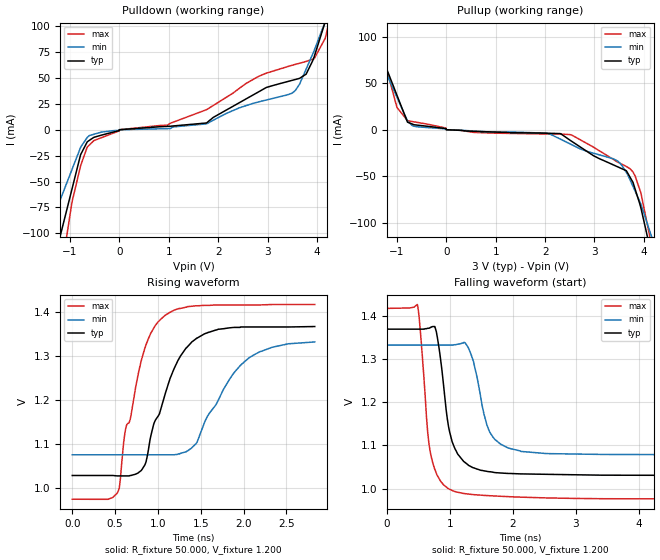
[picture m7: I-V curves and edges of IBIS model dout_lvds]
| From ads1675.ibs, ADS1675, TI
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|   dout_lvds Model
[Model]   dout_lvds
Model_type   Output
Polarity   Non-Inverting
Vmeas = 1.2
Vref = 1.2
Cref = 15pF
Rref = 50
|   typ   min   max
|   (nom PVT)   (Fast PVT)   (slow PVT)
|C_comp from frequency method(F=32MHz)
|Average
|C_comp   4.299e-12   3.477e-12   5.156e-12
|OFF state: BUFFER OUTPUT TURNED LOW
C_comp   5.050e-12   4.086e-12   5.984e-12
|ON state : BUFFER OUTPUT TURNED HIGH
|C_comp   3.549e-12   2.868e-12   4.327e-12
|C_comp from L-C Tank method(L=1nH)
|ON state : BUFFER OUTPUT TURNED HIGH
|Resonant Frequency(Hz)   2.67e9   2.90e9   2.54e9
|C_comp   3.557e-12   3.015e-12   3.930e-12
|OFF state: BUFFER OUTPUT TURNED LOW
|Resonant Frequency(Hz)   2.81e9   3.07e9   2.59e9
|C_comp   3.211e-12   2.690e-12   3.780e-12
| Where nom  PVT is Nominal Process,  3V,  51C
|   Fast PVT is Strong Process,   3.15V,  -40C
|   Slow PVT is Weak Process,   2.85V,  111C
[Voltage Range]   3   2.85   3.15
|Ambient Temperature   25   85   -40
|Junction Temperature
[Temperature Range]   51   111   -40
[Pullup Reference]   3   2.85   3.15
[Pulldown Reference]   0   0   0
[Power Clamp Reference]   3   2.85   3.15
[GND Clamp Reference]   0   0   0
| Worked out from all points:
|   slope of the pulldown table from 0 to 0.45 V, typ, clamps not added: 283 ohm
|   slope of the pullup table from 0 to 0.45 V, typ, clamps not added: 303 ohm
|   falling waveform, R_fixture 50.000, V_fixture 1.200: 20-80 % time 217ps typ, 254ps min, 171ps max; typ from 1.37 V to 1.03 V
|   rising waveform, R_fixture 50.000, V_fixture 1.200: 20-80 % time 365ps typ, 473ps min, 287ps max; typ from 1.03 V to 1.37 V
[Pulldown]
|   Voltage   I(typ)   I(min)   I(max)
-3V       -757.9mA   -626.3mA   -947.1mA
-1.605V   -208.1mA   -142mA     -302.5mA
-1.209V   -104.6mA   -68.97mA   -150mA
-960.7mV  -57.33mA   -38.47mA   -69.97mA
-786mV    -24.07mA   -17mA      -34.82mA
-607mV    -10.2mA    -5.593mA   -14.68mA
1.764V    6.534mA    5.696mA    19.39mA
3.471V    47.37mA    34.88mA    61.94mA
3.78V     53.67mA    58.53mA    65.96mA
4.167V    104.3mA    104.7mA    88.37mA
4.819V    202.8mA    186.8mA    220.7mA
6V        351mA      335.5mA    392.9mA
[Pullup]
|   Voltage   I(typ)   I(min)   I(max)
-3V       308.7mA    297.4mA    357.2mA
-1.956V   167.4mA    149.6mA    211.4mA
-998.6mV  37.09mA    34.98mA    23.98mA
-786mV    8.18mA     9.541mA    9.82mA
-692.5mV  6.225mA    4.63mA     8.872mA
2.032V    -3.754mA   -3.624mA   -4.613mA
2.52V     -11.82mA   -15.64mA   -5.368mA
3.468V    -39.92mA   -33.69mA   -34.84mA
3.78V     -56.75mA   -61.12mA   -45.58mA
3.945V    -85.4mA    -80.96mA   -69.36mA
4.193V    -143.8mA   -121.1mA   -134.3mA
6V        -766.8mA   -686.9mA   -881.5mA
[Ramp]
R_load = 50
|   typ   min   max
dV/dt_r   0.202758/3.64324e-10   0.145278/4.73067e-10   0.273559/2.87219e-10
dV/dt_f   0.204266/2.16563e-10   0.146447/2.48791e-10   0.273866/1.70953e-10
[Falling Waveform]
R_fixture = 50.000
V_fixture = 1.200
V_fixture_min = 1.200
V_fixture_max = 1.200
|  time   V(typ)   V(min)   V(max)
0s        1.369V     1.332V     1.417V
484ps     1.369V     1.332V     1.425V
648ps     1.371V     1.332V     1.128V
760ps     1.375V     1.332V     1.044V
976ps     1.145V     1.332V     999.9mV
1.084ns   1.091V     1.333V     993mV
1.332ns   1.051V     1.312V     986.7mV
1.64ns    1.039V     1.129V     983.4mV
2.124ns   1.034V     1.086V     980.2mV
10ns      1.029V     1.076V     975.1mV
[Rising Waveform]
R_fixture = 50.000
V_fixture = 1.200
V_fixture_min = 1.200
V_fixture_max = 1.200
|  time   V(typ)   V(min)   V(max)
0s        1.029V     1.076V     975.1mV
528ps     1.028V     1.076V     990mV
624ps     1.028V     1.076V     1.136V
676ps     1.029V     1.076V     1.156V
812ps     1.042V     1.076V     1.294V
1.088ns   1.216V     1.076V     1.393V
1.392ns   1.331V     1.091V     1.413V
1.54ns    1.35V      1.147V     1.415V
2.064ns   1.366V     1.296V     1.416V
2.832ns   1.367V     1.332V     1.417V
